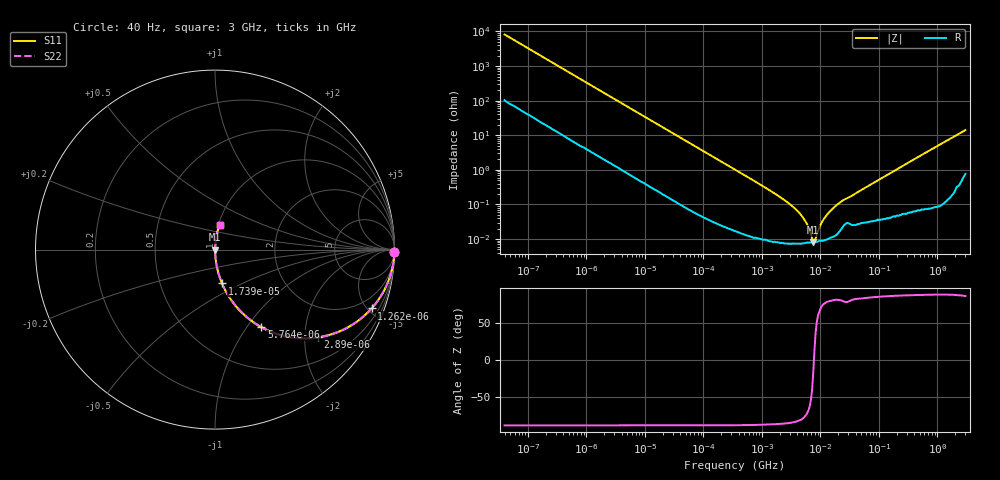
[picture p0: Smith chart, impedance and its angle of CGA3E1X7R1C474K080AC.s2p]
! S-parameter Generated by TDK Corporation
! Copyright(C) 2015 TDK Corporation.
! All Rights Reserved.
! TDK P/N: CGA3E1X7R1C474K080AC (Multilayer Ceramic Chip Capacitors)
! Property: C=470nF
! Size(LxWxT): 1.6x0.8x0.8mm, 0.063x0.031x0.031inches
! Model Type: s2p (Touchstone File Format Version 1.0)
! Frequency: DC=Yes Start=0.00004MHz Stop=3000MHz 396points Log-sweep
! Note: This model was converted from impedance.
! Model Generated on Jun. 23, 2015
! Hash(MD5):
! Port Assignments:
!  1 ---| |--- 2
! Applicable Conditions:
!  Temperature = 25 degC
!  DC Bias Voltage = 0 V
!  Small Signal Operation
! Terms and conditions regarding TDK Simulation Models
! (1)This simulation model is being provided solely for informational purposes. Please refer to the specifications of the products in terms of detailed characteristics of such products.
! (2)In no event shall TDK Corporation of any of its subsidiaries be liable for any loss or damage arising, directly or indirectly,
!  From any information contained in this simulation model, including, but not limited to loss or damages arising from any inaccuracies, omissions or errors in connection with such information.
! (3)Any and all copyrights on this simulation model are owned by TDK Corporation.
!  Duplication or redistribution of this simulation model without prior written permission from TDK Corporation is prohibited.
! (4)This simulation model is subject to any modification or change without any prior notice.
! (5)Neither TDK Corporation nor any of its subsidiaries shall make any warranty, express or implied,
!  Including but not limited to the correctness, implied warranties of merchantability and fitness for a particular purpose with respect to this simulation models.
! (6)The use of this simulation model shall be deemed to have consented to the terms and conditions hereof.
# MHz S MA R 50
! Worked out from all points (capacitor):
!   395 points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, 40 Hz to 3 GHz, reference 50 ohm
!   read as one part in series: C = 485 nF near 41.88 Hz
!   lowest |Z| = 8.11 mohm at 7.564 MHz (marker M1)
!   series resonance near 7.74 MHz, so ESL is about 870 pH
!   S11 on the Smith chart (normalised r, x): 40 Hz: open; 1.262 kHz: 1.06, -5.30; 2.89 kHz: 1.03, -2.33; 5.764 kHz: 1.01, -1.17; 17.39 kHz: 1.00, -0.39; 3 GHz: 1.02, +0.28
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4e-05  0.9998 -0.7  0.01219 88.6  0.01219 88.6  0.9998 -0.7
0.0002520917  0.9962 -4.3  0.07579 85.0  0.07579 85.0  0.9962 -4.3
0.000834128  0.9675 -14.0  0.2418 75.3  0.2418 75.3  0.9675 -14.0
0.001262176  0.932 -20.6  0.3515 68.7  0.3515 68.7  0.932 -20.6
0.002889976  0.7543 -40.4  0.6476 49.0  0.6476 49.0  0.7543 -40.4
0.005763764  0.5037 -59.1  0.858 30.2  0.858 30.2  0.5037 -59.1
0.009562432  0.3338 -69.8  0.9387 19.5  0.9387 19.5  0.3338 -69.8
0.01739424  0.1927 -78.2  0.979 11.1  0.979 11.1  0.1927 -78.2
0.05755453  0.06033 -85.9  0.9975 3.5  0.9975 3.5  0.06033 -85.9
0.3464102  0.01021 -88.5  0.9998 0.6  0.9998 0.6  0.01021 -88.5
1.581893  0.002171 -87.7  0.9999 0.1  0.9999 0.1  0.002171 -87.7
3.459106  0.0008347 -84.9  0.9999 0.0  0.9999 0.0  0.0008347 -84.9
4.5592  0.0005191 -81.9  0.9999 0.0  0.9999 0.0  0.0005191 -81.9
5.738865  0.0002935 -74.5  0.9999 0.0  0.9999 0.0  0.0002935 -74.5
7.22376  0.0001021 -39.4  0.9999 0.0  0.9999 0.0  0.0001021 -39.4
7.563987  8.109e-05 -14.7  0.9999 0.0  0.9999 0.0  8.109e-05 -14.7
8.293268  0.000105 38.1  0.9999 -0.0  0.9999 -0.0  0.000105 38.1
9.969551  0.0002538 69.4  0.9999 -0.0  0.9999 -0.0  0.0002538 69.4
11.44558  0.0003828 76.3  0.9999 -0.0  0.9999 -0.0  0.0003828 76.3
18.13479  0.000901 81.9  0.9999 -0.1  0.9999 -0.1  0.000901 81.9
150.6385  0.007816 86.5  0.9996 -0.4  0.9996 -0.4  0.007816 86.5
3000  0.1392 78.9  0.9828 -8.0  0.9828 -8.0  0.1392 78.9
